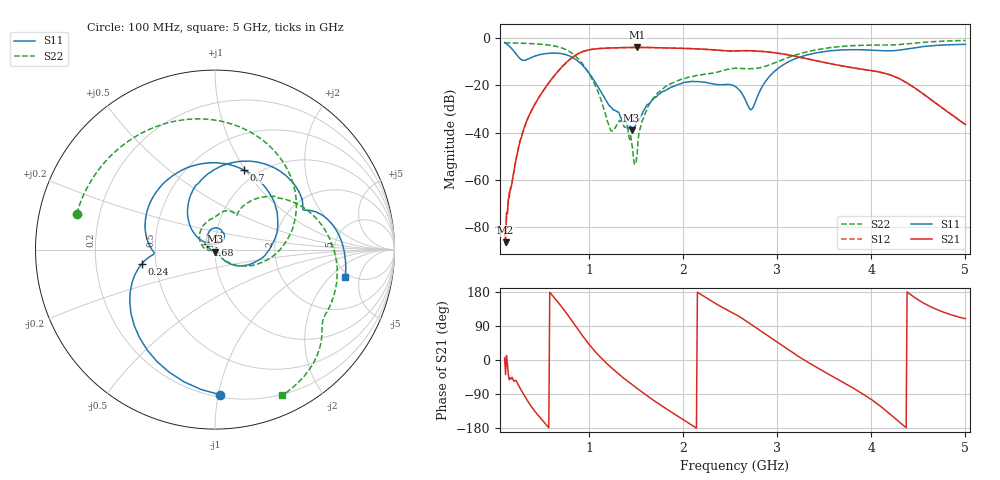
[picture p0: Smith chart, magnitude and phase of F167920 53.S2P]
!  2-Port S-parameters saved by WinCal
! VAR MeasName=S-Parameters (CALIBRATED_DATA) read from VNA (N5242A)
! VAR MeasDate=2016-11-22 9:58:08
! VAR NAME=F167920 53
! VAR FILENAME=F167920 53.S2P
! VAR DATE=2016-11-22 9:58:08
! VAR PHYS_PORTS=1,2
# Hz S DB R 50
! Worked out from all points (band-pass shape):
!   491 points, 100 MHz to 5 GHz, reference 50 ohm
!   highest |S21| = -3.89 dB at 1.51 GHz (marker M1); lowest = -86.3 dB at 110 MHz (marker M2)
!   |S21| within 3 dB of the highest: 868.3 MHz to 3.092 GHz (2.224 GHz wide, 112 % of centre)
!   lowest |S11| = -38.9 dB at 1.45 GHz (marker M3), VSWR 1.02, Z = 49.9 - j1.12 ohm
!   |S11| at or under -10 dB: 888 MHz to 3.118 GHz (2.23 GHz wide, 111 % of centre)
!   |S22| runs from -53.3 to -1.0 dB; largest |S21 - S12| = 0.0015
!   S11 on the Smith chart (normalised r, x): 100 MHz: 0.22, -1.01; 240 MHz: 0.42, -0.08; 700 MHz: 0.87, +0.99; 1.68 GHz: 0.92, +0.05; 5 GHz: 4.57, -3.10
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1e8  -1.84 -88.0  -80.54 5.5  -81.17 74.5  -1.98 165.5
1.1e8  -2.12 -95.7  -86.25 -38.2  -87.91 106.1  -1.99 164.0
1.7e8  -4.18 -136.7  -62.89 -50.3  -63.24 -46.3  -2.03 155.2
2.4e8  -7.61 -168.9  -47.85 -64.0  -47.85 -62.0  -2.09 144.8
4e8  -7.94 165.3  -29.47 -128.2  -29.48 -127.9  -2.34 119.1
7e8  -6.51 69.8  -12.55 142.6  -12.56 142.5  -4.03 55.3
9.2e8  -11.04 -6.7  -5.86 67.2  -5.85 67.3  -10.45 -10.7
1.22e9  -28.78 -43.3  -4.16 -16.9  -4.16 -16.9  -38.22 -13.3
1.34e9  -33.81 -44.7  -3.99 -42.5  -3.99 -42.5  -35.29 42.6
1.45e9  -38.95 -93.5  -3.93 -63.9  -3.93 -63.9  -44.00 37.2
1.49e9  -37.11 -135.2  -3.91 -71.3  -3.91 -71.4  -53.34 140.6
1.51e9  -35.22 -159.9  -3.89 -75.2  -3.88 -75.2  -48.93 -165.9
1.55e9  -32.76 -179.9  -3.91 -82.6  -3.90 -82.5  -37.05 -167.0
1.68e9  -25.83 145.8  -3.99 -105.6  -3.98 -105.6  -25.42 175.1
1.74e9  -23.72 135.5  -4.04 -115.7  -4.04 -115.8  -22.77 163.6
2.11e9  -18.30 85.8  -4.45 -175.0  -4.46 -175.0  -16.07 109.2
2.55e9  -20.35 56.6  -5.41 121.2  -5.41 121.2  -12.73 67.9
2.72e9  -30.26 95.5  -5.34 94.3  -5.33 94.3  -12.93 57.8
2.97e9  -14.02 135.4  -6.17 51.9  -6.16 51.8  -10.46 56.4
3.37e9  -6.56 85.0  -9.16 -12.6  -9.16 -12.7  -5.27 25.6
4.19e9  -5.36 24.3  -15.41 -140.9  -15.43 -140.8  -2.90 -32.2
5e9  -2.60 -11.9  -36.48 109.4  -36.48 109.6  -0.97 -65.1
